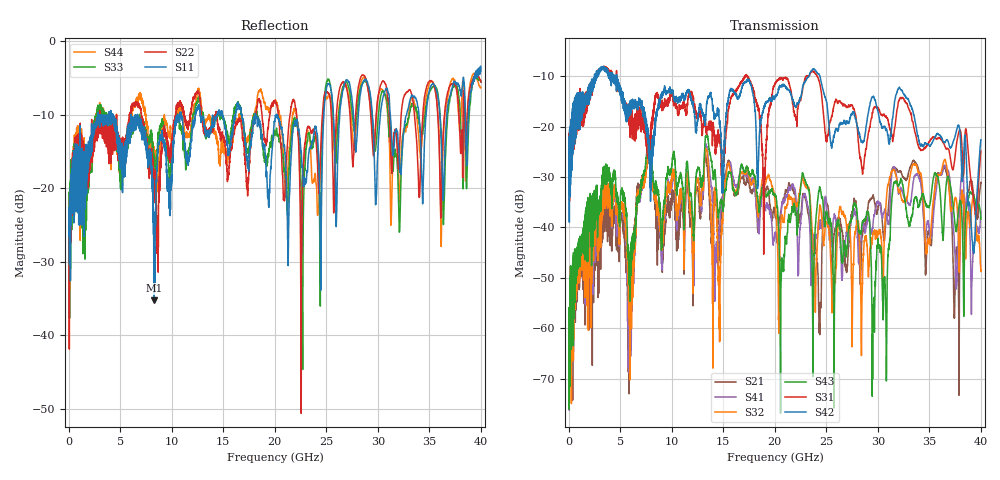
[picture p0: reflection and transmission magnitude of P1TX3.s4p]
!Agilent Technologies,N5245A,MY49151084,A.09.20.08
!Agilent N5245A: A.09.20.08
!Date: Thursday, March 01, 2012 14:05:35
!Correction: S11(Full 4 Port(1,2,3,4))
!S12(Full 4 Port(1,2,3,4))
!S13(Full 4 Port(1,2,3,4))
!S14(Full 4 Port(1,2,3,4))
!S21(Full 4 Port(1,2,3,4))
!S22(Full 4 Port(1,2,3,4))
!S23(Full 4 Port(1,2,3,4))
!S24(Full 4 Port(1,2,3,4))
!S31(Full 4 Port(1,2,3,4))
!S32(Full 4 Port(1,2,3,4))
!S33(Full 4 Port(1,2,3,4))
!S34(Full 4 Port(1,2,3,4))
!S41(Full 4 Port(1,2,3,4))
!S42(Full 4 Port(1,2,3,4))
!S43(Full 4 Port(1,2,3,4))
!S44(Full 4 Port(1,2,3,4))
!S4P File: Measurements: <S11,S12,S13,S14>,
!<S21,S22,S23,S24>,
!<S31,S32,S33,S34>,
!<S41,S42,S43,S44>:
# Hz S  dB  R 50
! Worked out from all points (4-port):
!   3996 points, 50 MHz to 40 GHz, reference 50 ohm
!   strongest paths, dB at 50 MHz, 10.04 GHz, 20.03 GHz, 30.02 GHz, 40 GHz:
!     S42: -25.0, -12.9, -14.2, -17.0, -22.6
!     S31: -25.3, -13.5, -11.5, -16.4, -24.8
!     S43: -59.1, -27.4, -33.5, -42.2, -38.4
!     S32: -62.2, -29.9, -34.7, -41.4, -48.5
!     S41: -61.4, -31.2, -41.5, -35.0, -36.8
!     S21: -60.2, -33.7, -37.5, -36.1, -31.2
!   lowest |S11| = -35.3 dB at 8.31 GHz (marker M1), VSWR 1.04, Z = 51.6 + j0.654 ohm
!   |S11| at or under -10 dB: start of sweep to 2.876 GHz; 6.68 GHz to 10.78 GHz (4.102 GHz wide, 47 % of centre); 20.18 GHz to 24.76 GHz (4.577 GHz wide, 20.4 % of centre)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
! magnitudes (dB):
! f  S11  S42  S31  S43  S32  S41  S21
! 50 MHz  -24.4  -25.0  -25.3  -59.1  -62.2  -61.4  -60.2
! 8.31 GHz  -35.3  -21.7  -16.4  -32.2  -33.4  -33.3  -33.1
! 24.35 GHz  -19.4  -9.8  -11.3  -31.9  -36.0  -40.1  -59.0
! 29.58 GHz  -13.0  -14.0  -16.4  -59.4  -41.2  -38.3  -33.9
! 31.68 GHz  -12.3  -14.4  -19.8  -30.9  -29.3  -28.4  -28.4
! 39.26 GHz  -5.2  -44.0  -34.1  -33.6  -34.2  -45.0  -32.9
! 40 GHz  -4.1  -22.6  -24.8  -38.4  -48.5  -36.8  -31.2
